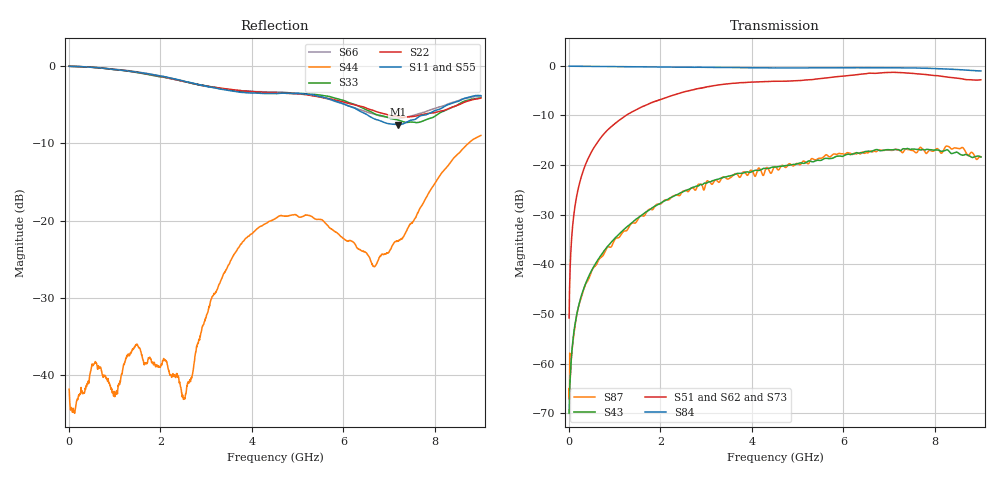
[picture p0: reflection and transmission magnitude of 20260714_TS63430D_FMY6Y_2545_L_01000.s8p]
# GHz S DB R 50
! CMT, SN0916, 25263762, 26.7.0
! Date: 15.07.2026 14:55:46
! Data: Format
! Freq S1.1:dB/Ang S1.2:dB/Ang S1.3:dB/Ang S1.4:dB/Ang S1.5:dB/Ang S1.6:dB/Ang S1.7:dB/Ang S1.8:dB/Ang
!  S2.1:dB/Ang S2.2:dB/Ang S2.3:dB/Ang S2.4:dB/Ang S2.5:dB/Ang S2.6:dB/Ang S2.7:dB/Ang S2.8:dB/Ang
!  S3.1:dB/Ang S3.2:dB/Ang S3.3:dB/Ang S3.4:dB/Ang S3.5:dB/Ang S3.6:dB/Ang S3.7:dB/Ang S3.8:dB/Ang
!  S4.1:dB/Ang S4.2:dB/Ang S4.3:dB/Ang S4.4:dB/Ang S4.5:dB/Ang S4.6:dB/Ang S4.7:dB/Ang S4.8:dB/Ang
!  S5.1:dB/Ang S5.2:dB/Ang S5.3:dB/Ang S5.4:dB/Ang S5.5:dB/Ang S5.6:dB/Ang S5.7:dB/Ang S5.8:dB/Ang
!  S6.1:dB/Ang S6.2:dB/Ang S6.3:dB/Ang S6.4:dB/Ang S6.5:dB/Ang S6.6:dB/Ang S6.7:dB/Ang S6.8:dB/Ang
!  S7.1:dB/Ang S7.2:dB/Ang S7.3:dB/Ang S7.4:dB/Ang S7.5:dB/Ang S7.6:dB/Ang S7.7:dB/Ang S7.8:dB/Ang
!  S8.1:dB/Ang S8.2:dB/Ang S8.3:dB/Ang S8.4:dB/Ang S8.5:dB/Ang S8.6:dB/Ang S8.7:dB/Ang S8.8:dB/Ang
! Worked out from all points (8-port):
!   2001 points, 10 MHz to 9 GHz, reference 50 ohm
!   strongest paths, dB at 10 MHz, 2.257 GHz, 4.505 GHz, 6.753 GHz, 9 GHz:
!     S84: -0.1, -0.3, -0.4, -0.4, -1.0
!     S51: -50.8, -6.0, -3.1, -1.5, -2.8
!     S62: -51.1, -5.9, -3.3, -1.8, -2.7
!     S73: -51.3, -6.1, -3.3, -1.7, -2.8
!     S43: -70.0, -26.4, -20.4, -16.9, -18.4
!     S87: -67.0, -26.4, -20.3, -17.0, -18.3
!   lowest |S11| = -7.6 dB at 7.184 GHz (marker M1), VSWR 2.43, Z = 21.4 - j9.39 ohm
!   |S11| at or under -10 dB: nowhere
